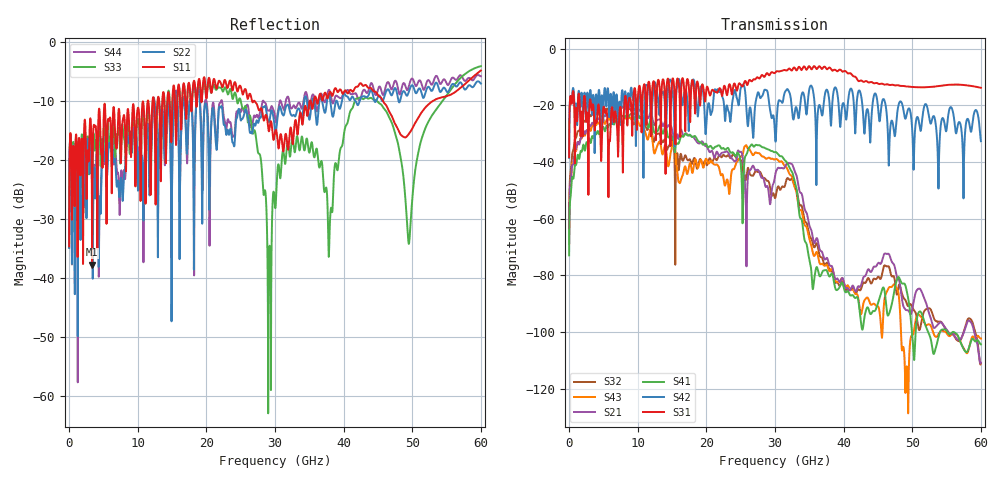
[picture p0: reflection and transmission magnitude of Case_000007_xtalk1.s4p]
! Info: Touchstone file created by circ.  Input file=CasetestDOE_NRZ_template_000007.circ
# Hz S RI R 50
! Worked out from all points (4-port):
!   6000 points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, 10 MHz to 60 GHz, reference 50 ohm
!   strongest paths, dB at 10 MHz, 15.01 GHz, 30.01 GHz, 45.01 GHz, 60 GHz:
!     S31: -38.3, -11.4, -8.5, -12.3, -13.8
!     S42: -38.5, -13.1, -30.5, -20.6, -32.6
!     S41: -72.9, -31.5, -36.5, -89.8, -104.3
!     S21: -68.6, -28.8, -44.8, -75.7, -110.7
!     S43: -68.9, -34.1, -39.0, -90.9, -102.3
!     S32: -65.2, -31.1, -52.7, -80.5, -110.9
!   lowest |S11| = -37.7 dB at 3.36 GHz (marker M1), VSWR 1.03, Z = 49.4 - j1.14 ohm
!   |S11| at or under -10 dB: start of sweep to 11.45 GHz; 27.08 GHz to 35.06 GHz (7.985 GHz wide, 25.7 % of centre); 45.76 GHz to 52.92 GHz (7.159 GHz wide, 14.5 % of centre)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
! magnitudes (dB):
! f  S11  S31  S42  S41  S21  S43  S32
! 10 MHz  -34.6  -38.3  -38.5  -72.9  -68.6  -68.9  -65.2
! 3.36 GHz  -37.7  -21.1  -22.3  -30.9  -26.2  -27.2  -23.1
! 24.18 GHz  -6.8  -12.6  -14.7  -37.7  -39.7  -41.6  -37.9
! 29.2 GHz  -14.7  -9.3  -20.2  -35.7  -53.6  -38.5  -47.7
! 35.58 GHz  -10.6  -6.4  -15.3  -84.2  -67.5  -72.6  -69.5
! 49.51 GHz  -15.5  -13.4  -21.1  -89.5  -92.6  -112.1  -90.6
! 60 GHz  -4.8  -13.8  -32.6  -104.3  -110.7  -102.3  -110.9
